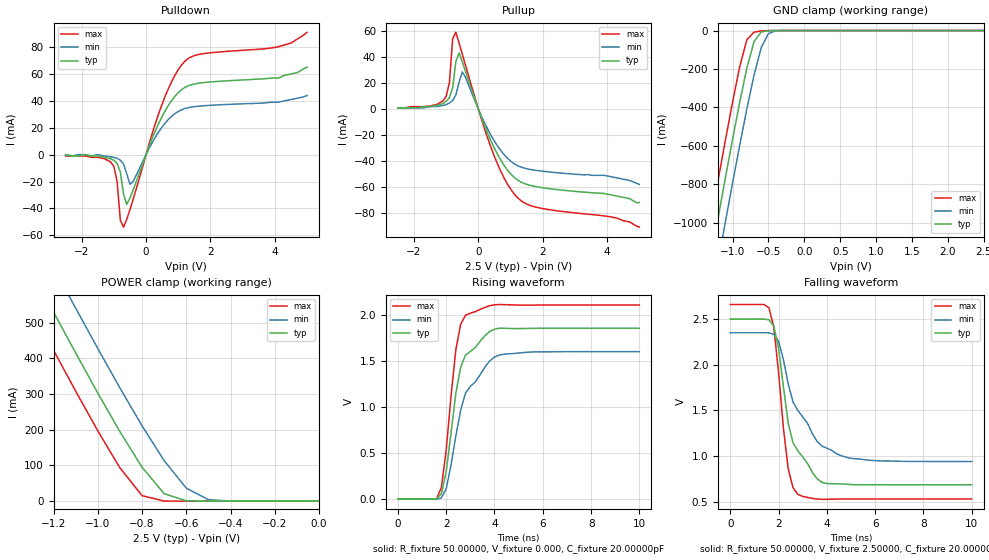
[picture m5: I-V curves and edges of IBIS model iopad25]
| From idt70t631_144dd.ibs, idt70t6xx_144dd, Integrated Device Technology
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|   Model iopad25
[Model]   iopad25
Model_type   I/O
Polarity   Non-Inverting
Enable   Active-Low
Vinl =  0.70000V
Vinh =  1.70000V
Vmeas =  1.25000V
C_comp   4.50000pF   4.50000pF   4.50000pF
[Temperature Range]   25.00000   100.00000   -40.00000
[Voltage Range]   2.50000V   2.30000V   2.70000V
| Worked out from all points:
|   slope of the pulldown table from 0 to 0.375 V, typ, clamps not added: 16.8 ohm
|   slope of the pullup table from 0 to 0.375 V, typ, clamps not added: 15.9 ohm
|   GND clamp passes 1 mA (typ) near -0.50 V on its own axis
|   POWER clamp passes 1 mA (typ) near -0.60 V on its own axis
|   rising waveform, R_fixture 50.00000, V_fixture 0.000, C_fixture 20.00000pF: 20-80 % time 646ps typ, 1.07ns min, 500ps max; typ from 0 V to 1.85 V
|   falling waveform, R_fixture 50.00000, V_fixture 2.50000, C_fixture 20.00000pF: 20-80 % time 804ps typ, 1.26ns min, 483ps max; typ from 2.5 V to 0.687 V
[Pulldown]
| voltage   I(typ)   I(min)   I(max)
-2.5V     0A         0A         -1mA
-1.1V     -3.1mA     -1.6mA     -5.4mA
-1V       -4.2mA     -2.1mA     -8.8mA
-900mV    -6.6mA     -2.8mA     -19.8mA
-800mV    -12.8mA    -4.1mA     -48.76mA
-700mV    -29.43mA   -7mA       -53.96mA
-600mV    -37.03mA   -14.17mA   -48.13mA
-500mV    -32.29mA   -22.11mA   -40.89mA
500mV     28.49mA    20.63mA    37.7mA
1.2V      49.93mA    34.24mA    69.32mA
4.1V      56.9mA     39mA       80.2mA
5V        65mA       44mA       91mA
[Pullup]
| voltage   I(typ)   I(min)   I(max)
-2.5V     1mA        1mA        1mA
-1.1V     4.3mA      2.9mA      6.4mA
-900mV    8.9mA      4.8mA      20.66mA
-800mV    16.52mA    6.6mA      54.26mA
-700mV    36.86mA    11mA       59.33mA
-600mV    43.46mA    20.89mA    50.96mA
-500mV    36.57mA    28.78mA    42.4mA
400mV     -24.99mA   -20.52mA   -30.09mA
800mV     -43.39mA   -35.12mA   -53.17mA
1.2V      -54.33mA   -43.34mA   -67.83mA
1.8V      -59.77mA   -47.2mA    -75.63mA
5V        -72mA      -58mA      -91mA
[GND_clamp]
| voltage   I(typ)   I(min)   I(max)
-2.5V     -3.74A     -3.961A    -3.553A
-1.4V     -1.389A    -1.618A    -1.194A
-1.3V     -1.179A    -1.409A    -984.4mA
-1.2V     -972.3mA   -1.201A    -776.5mA
-1.1V     -767.3mA   -996.6mA   -571.8mA
-900mV    -372.8mA   -596.6mA   -188mA
-800mV    -194.3mA   -406.4mA   -47.16mA
-700mV    -57.22mA   -230.7mA   -8.4mA
-600mV    -7.393mA   -88.33mA   -2.169mA
-500mV    -1.009mA   -16.09mA   -229.2uA
-400mV    -92.71uA   -1.476mA   -9.663uA
2.5V      510.3pA    625.2nA    1.837pA
[POWER_clamp]
| voltage   I(typ)   I(min)   I(max)
-2.5V     2.074A     2.195A     1.972A
-1.4V     762.2mA    887.1mA    656mA
-1.3V     645.3mA    770.5mA    538.7mA
-1.2V     529.4mA    654.8mA    422.5mA
-1.1V     414.9mA    540.2mA    308mA
-1V       302.5mA    427.3mA    196.9mA
-900mV    194.4mA    316.8mA    93.14mA
-800mV    94.88mA    210.9mA    15.33mA
-700mV    20.78mA    113.2mA    204uA
-600mV    865.9uA    36.42mA    1.94uA
-500mV    23.06uA    3.99mA     31.75nA
0V        510.3pA    46.37nA    1.886pA
[Ramp]
| variable   typ   min   max
dV/dt_r   1.11300/0.34369n   0.96060/0.43779n   1.26420/0.27148n
dV/dt_f   1.08936/0.31359n   0.87954/0.39756n   1.27392/0.24900n
R_load = 50.00000
[Rising Waveform]
R_fixture = 50.00000
V_fixture = 0.000
C_fixture = 20.00000pF
R_dut = 0.11800
L_dut = 6.90000nH
C_dut = 1.23000pF
| time   V(typ)   V(min)   V(max)
0s        0V         0V         0V
1.6ns     594.5uV    -1.623mV   3.103mV
1.8ns     58.84mV    12.68mV    127.1mV
2ns       301.7mV    113.9mV    533.4mV
2.4ns     1.149V     687.3mV    1.622V
2.6ns     1.431V     965.8mV    1.896V
2.8ns     1.561V     1.15V      1.992V
3.8ns     1.816V     1.497V     2.096V
4.2ns     1.851V     1.562V     2.109V
10ns      1.852V     1.598V     2.103V
[Falling Waveform]
R_fixture = 50.00000
V_fixture = 2.50000
C_fixture = 20.00000pF
R_dut = 0.11800
L_dut = 6.90000nH
C_dut = 1.23000pF
| time   V(typ)   V(min)   V(max)
0s        2.5V       2.351V     2.66V
1.6ns     2.494V     2.35V      2.625V
1.8ns     2.426V     2.333V     2.42V
2ns       2.183V     2.259V     1.921V
2.2ns     1.763V     2.061V     1.312V
2.4ns     1.361V     1.791V     862mV
2.8ns     1.058V     1.5V       582.2mV
3.8ns     713.3mV    1.11V      528mV
4.8ns     692.9mV    988.5mV    531.6mV
10ns      687.2mV    941.2mV    531.2mV
